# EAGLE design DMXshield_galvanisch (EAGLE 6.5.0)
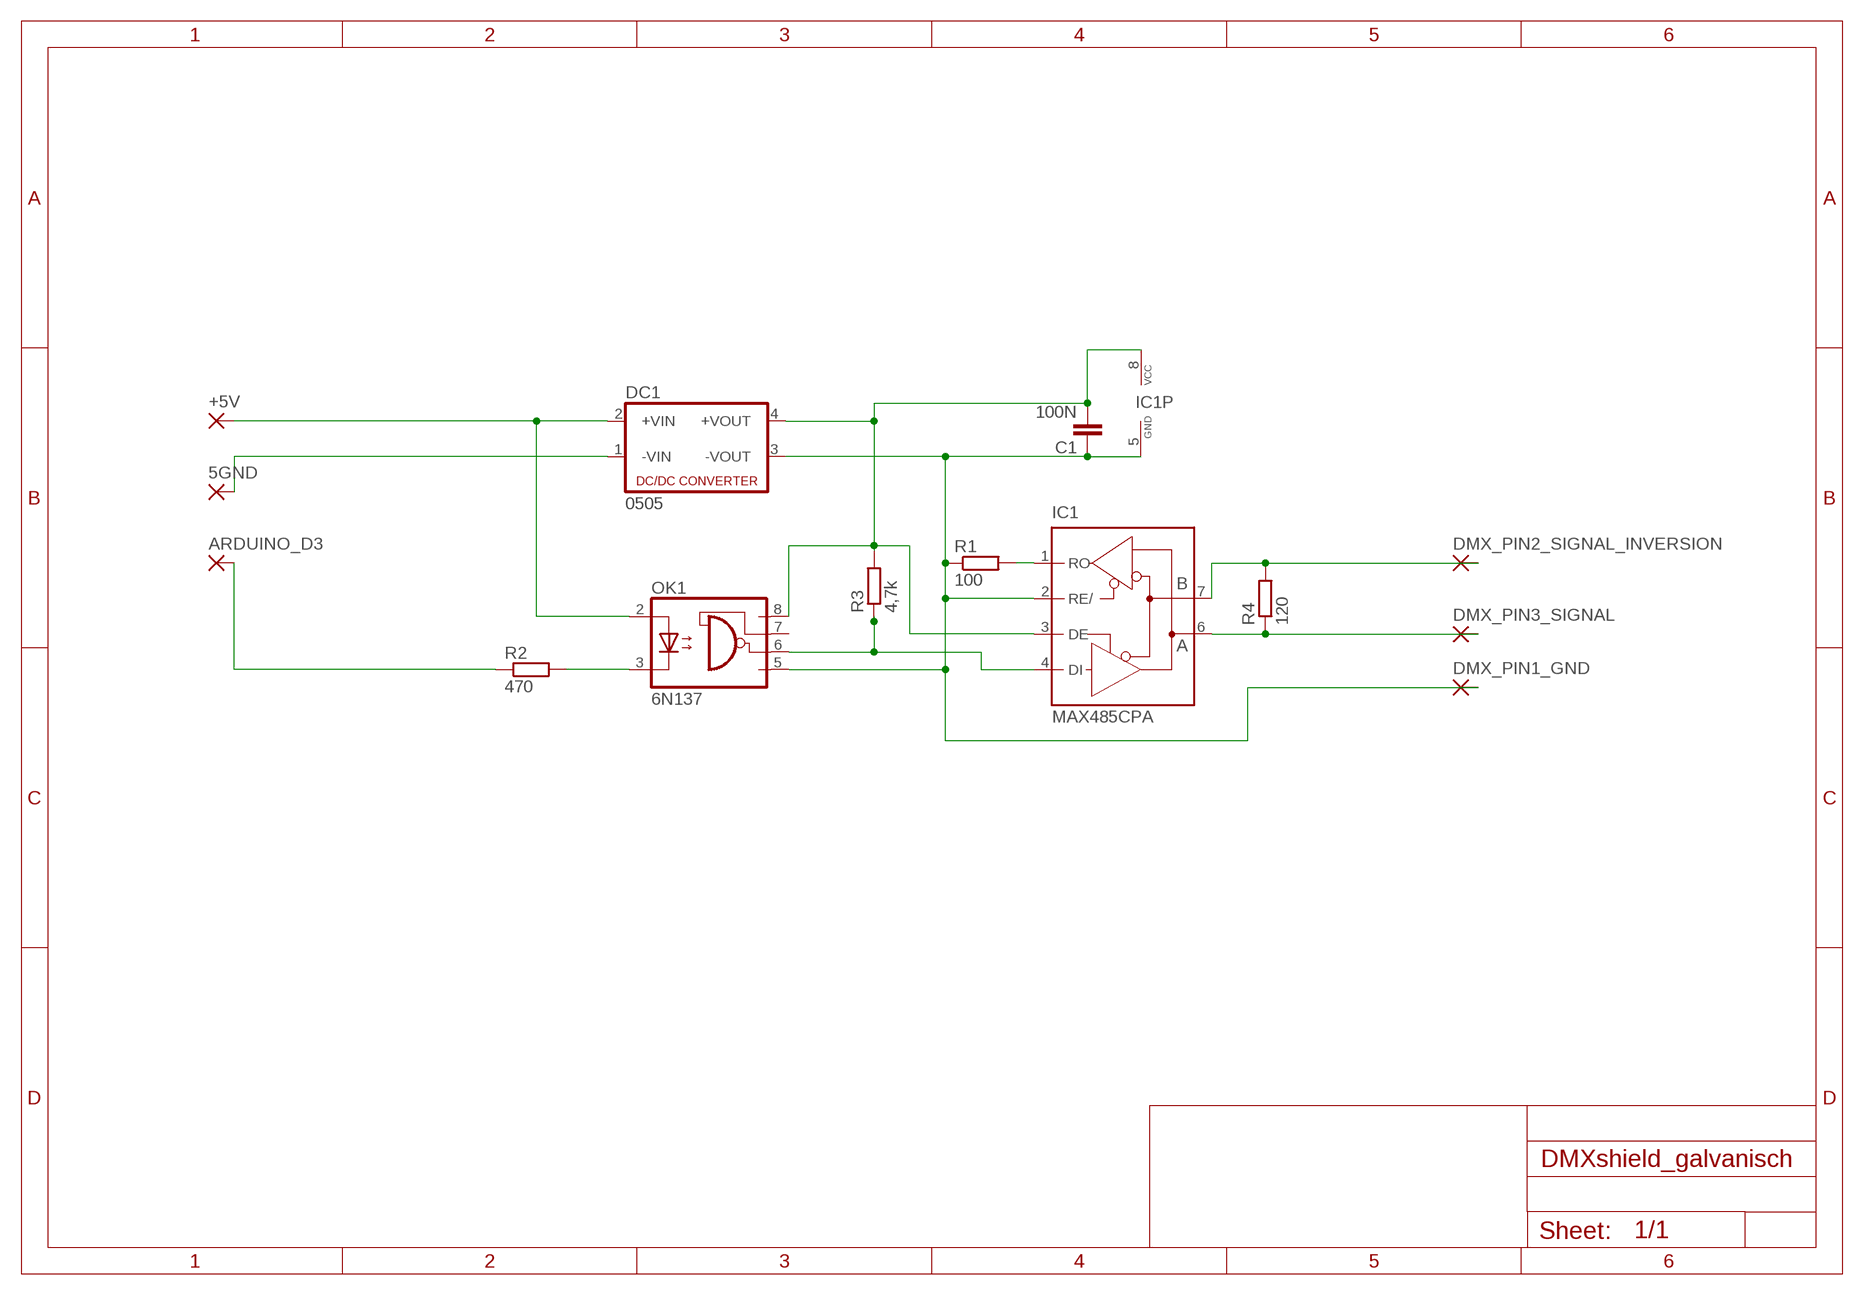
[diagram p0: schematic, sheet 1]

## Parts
5GND  3,81/1,4  [3,81/1,4]
+5V  3,81/1,4  [3,81/1,4]
ARDUINO_D3  3,81/1,4  [3,81/1,4]
C1  100N  C-EUC1206  [C1206]
DC1  0505  NME  [NME]
DMX_PIN1_GND  2,54/1,1  [2,54/1,1]
DMX_PIN2_SIGNAL_INVERSION  2,54/1,1  [2,54/1,1]
DMX_PIN3_SIGNAL  2,54/1,1  [2,54/1,1]
IC1  MAX485CPA  MAX481CPA  [DIL08]
OK1  6N137  [DIL08]
R1  100  R-EU_M1206  [M1206]
R2  470  R-EU_M1206  [M1206]
R3  4,7k  R-EU_M1206  [M1206]
R4  120  R-EU_M1206  [M1206]

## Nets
N$19: C1.2 DC1.4(+VOUT) IC1.3(DE) IC1.8(VCC) OK1.8(VCC) R3.2
N$21: +5V.1(P) DC1.2(+VIN) OK1.2(A)
N$32: IC1.1(RO) R1.2
N$33: 5GND.1(P) DC1.1(-VIN)
N$34: IC1.4(DI) OK1.6(VO) R3.1
N$35: ARDUINO_D3.1(P) R2.1
N$36: DMX_PIN3_SIGNAL.1(P) IC1.6(A) R4.1
N$37: DMX_PIN2_SIGNAL_INVERSION.1(P) IC1.7(B) R4.2
N$39: C1.1 DC1.3(-VOUT) DMX_PIN1_GND.1(P) IC1.2(RE/) IC1.5(GND) OK1.5(GND) R1.1
N$41: OK1.3(C) R2.2
Unconnected: OK1.7(VE)

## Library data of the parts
5GND +5V ARDUINO_D3 = wirepad:3,81/1,4: THROUGH-HOLE PAD
C1 = rcl:C-EU: CAPACITOR, European symbol
DC1 = dc-dc-converter:NME: DC-DC CONVERTER; MF: C & D TECHNOLOGIES, INC; MPN: NME1205D; OC_FARNELL: 1021466; OC_NEWARK: 98B8198
DMX_PIN1_GND DMX_PIN2_SIGNAL_INVERSION DMX_PIN3_SIGNAL = wirepad:2,54/1,1: THROUGH-HOLE PAD
IC1 = maxim:MAX481CPA: RS485 TRANSEIVER; MPN: MAX481CPA+; OC_FARNELL: unknown; OC_NEWARK: 99K3445
OK1 = optocoupler:6N137: MOTOROLA OPTO COUPLER; MPN: 6N137; OC_FARNELL: 1328376; OC_NEWARK: 52M1895
R1-R4 = rcl:R-EU_: RESISTOR, European symbol

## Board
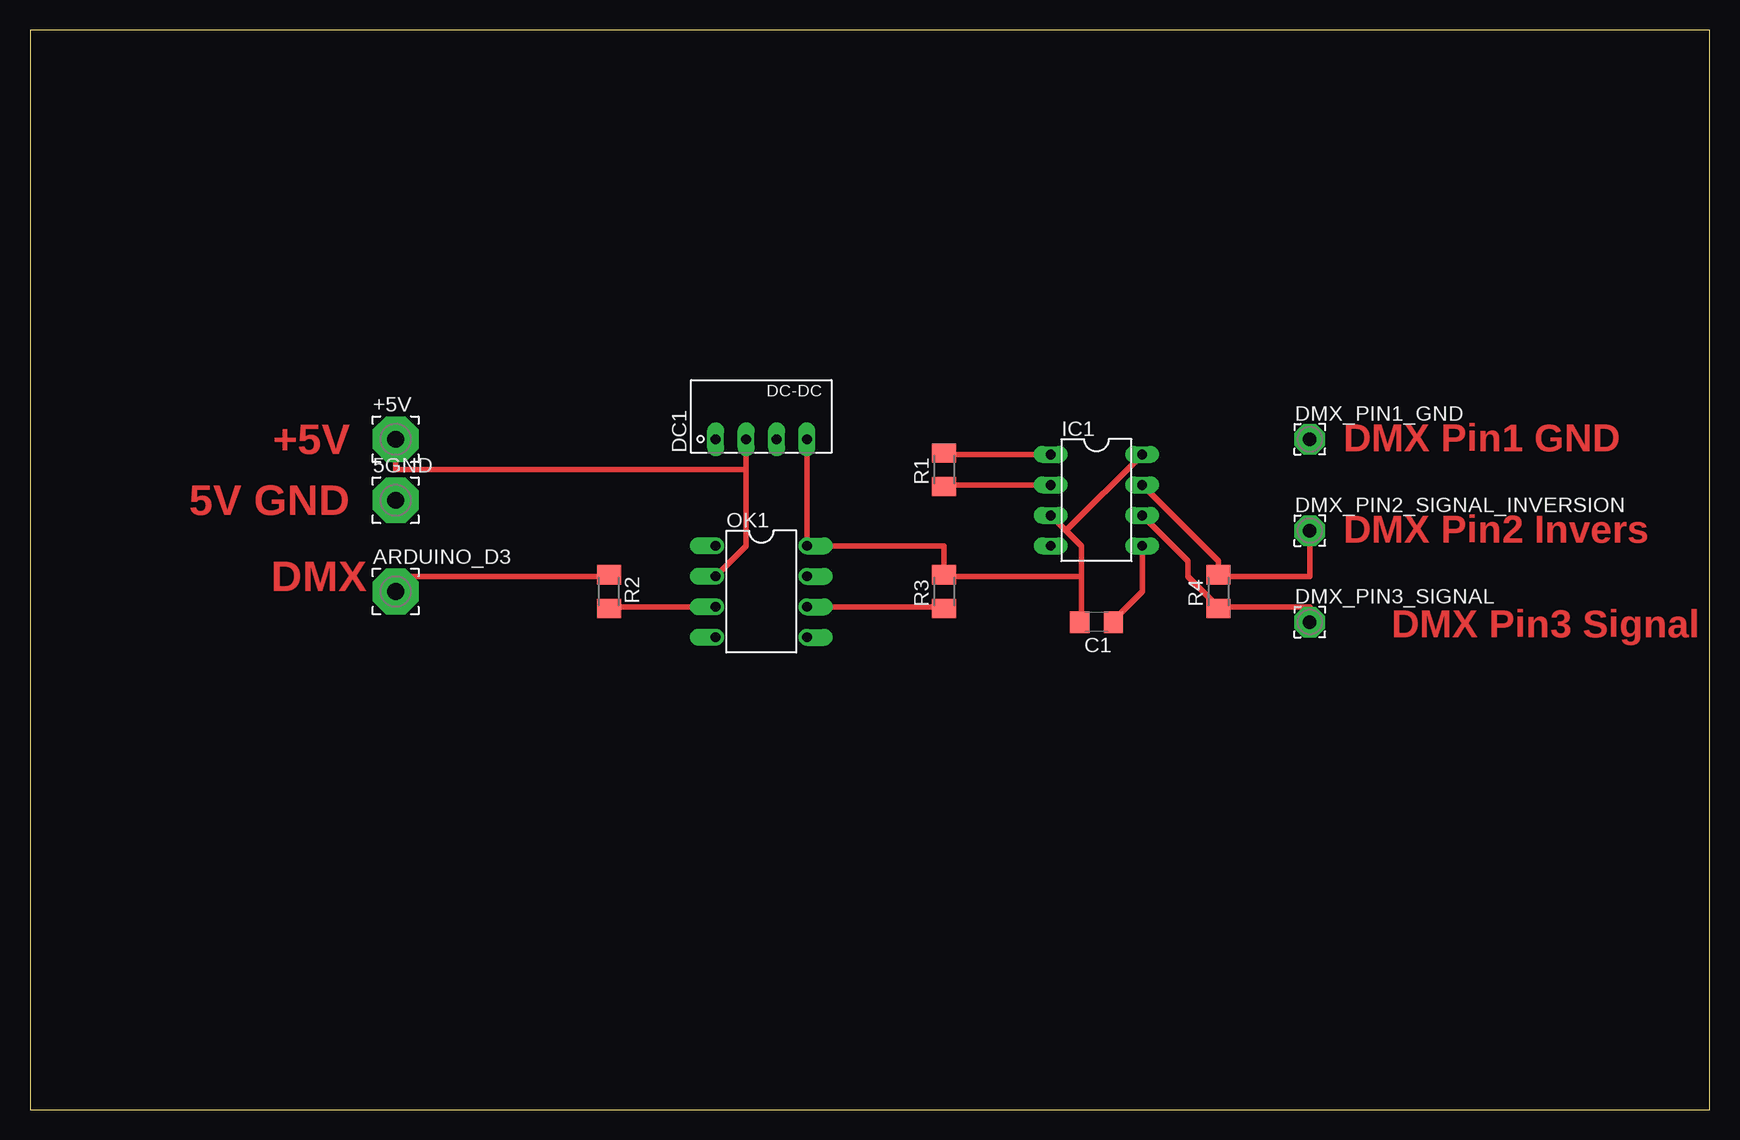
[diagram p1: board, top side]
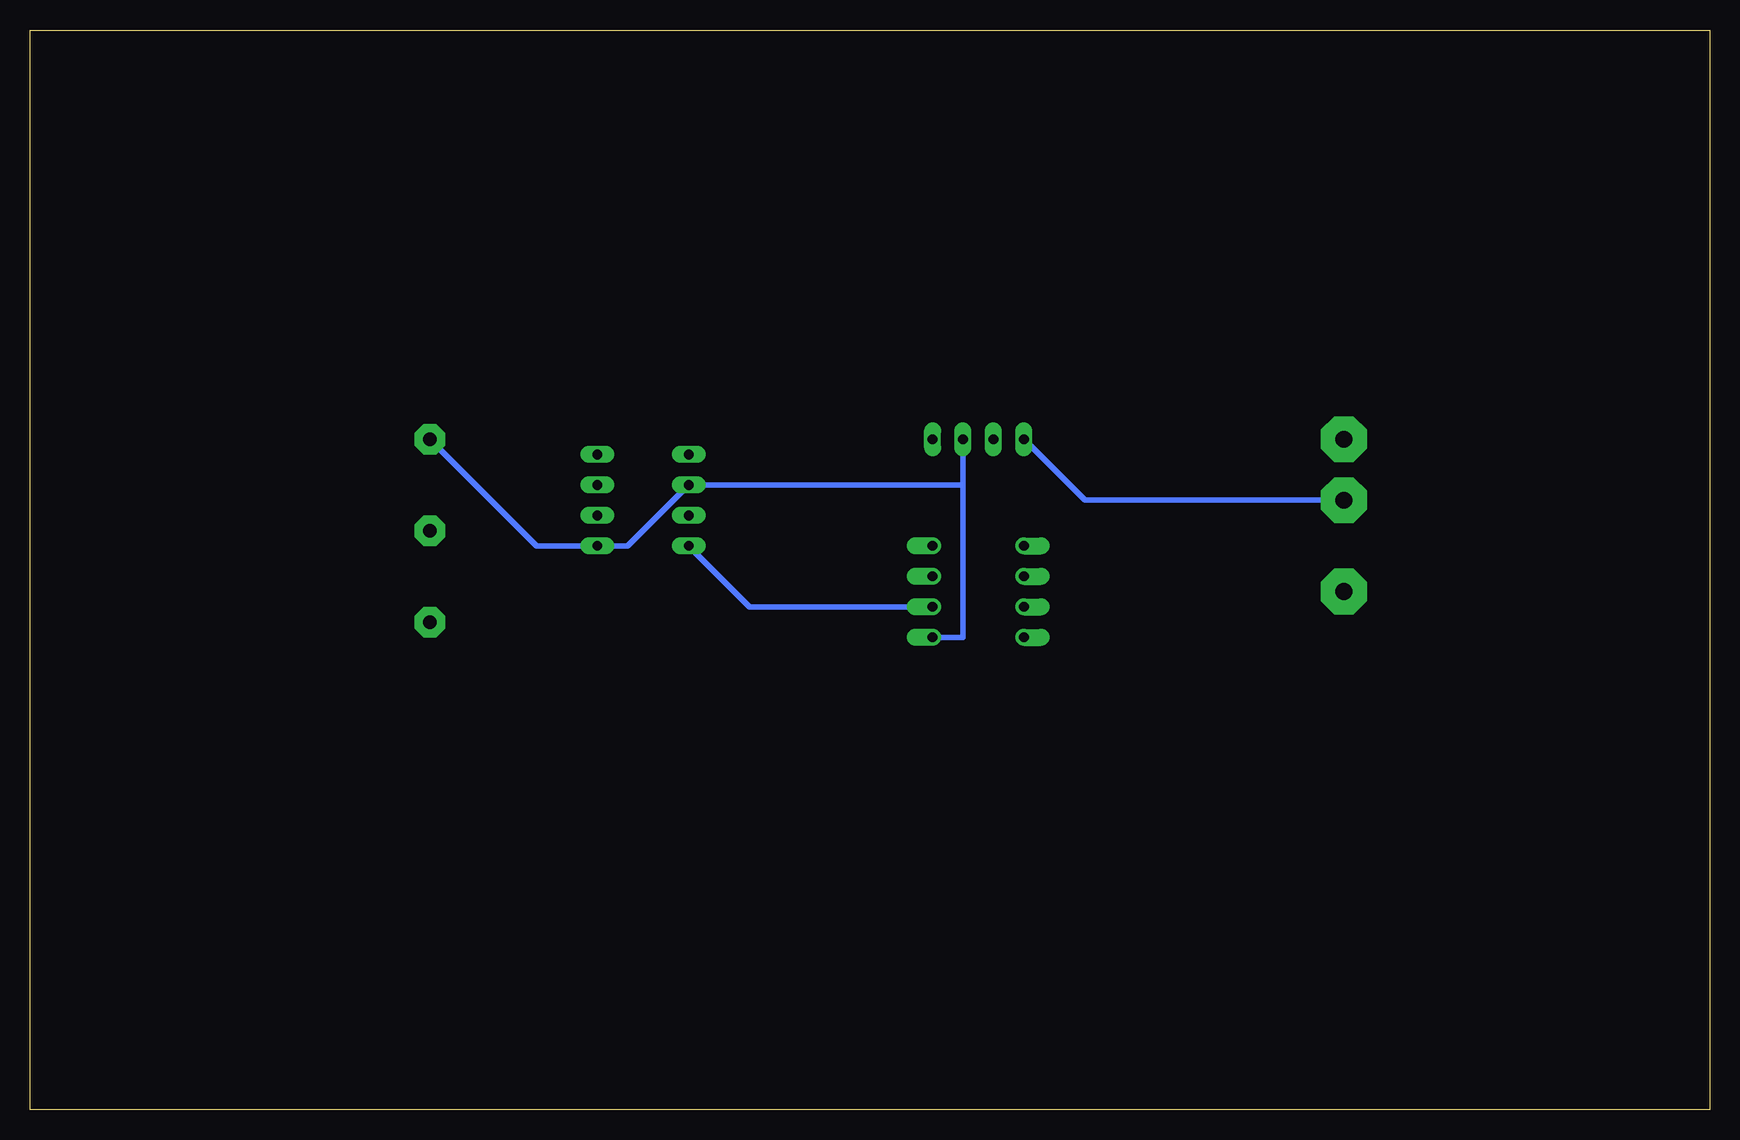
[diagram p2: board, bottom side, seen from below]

Size 140 x 90 mm. Coordinates in mm from the lower left corner, seen from the top.
Outline: 0,0 140,0 140,90 0,90 0,0
Copper layers (1*16): Top 0.035mm / dielectric 1.5mm / Bottom 0.035mm
Design rules "HTWG Sinnvoll *": minimum track width 18mil, minimum drill 0.4mm, track to track 12mil, track to pad 12mil, pad to pad 18mil, via to via 18mil, smd to smd 18mil, copper to edge 40mil, drill to drill 8mil, minimum pad ring 12mil, minimum via ring 20mil, stop-mask expansion 4mil, vias tented up to drill 0mil, thermal gap 10mil

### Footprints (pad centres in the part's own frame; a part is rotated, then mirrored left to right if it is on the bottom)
3,81/1,4 = drill 1.397 pad 3.81 octagon: 1 0,0
C1206 = smd 1.6 x 1.8: 1 -1.4,0; 2 1.4,0
NME = drill 0.813 long: 1 0,3.81; 2 0,1.27; 3 0,-1.27; 4 0,-3.81
2,54/1,1 = drill 1.118 pad 2.54 octagon: 1 0,0
DIL08 = drill 0.813 long: 1 -3.81,-3.81; 2 -1.27,-3.81; 3 1.27,-3.81; 4 3.81,-3.81; 5 3.81,3.81; 6 1.27,3.81; 7 -1.27,3.81; 8 -3.81,3.81
DIL08' = drill 0.813 offset: 1 -3.81,-3.81; 2 -1.27,-3.81; 3 1.27,-3.81; 4 3.81,-3.81; 5 3.81,3.81; 6 1.27,3.81; 7 -1.27,3.81; 8 -3.81,3.81
M1206 = smd 1.6 x 2: 1 -1.4,0; 2 1.4,0

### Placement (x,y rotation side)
5GND  30.48,50.8 0 top
+5V  30.48,55.88 0 top
ARDUINO_D3  30.48,43.18 0 top
C1  88.9,40.64 180 top
DC1  60.96,55.88 90 top
DMX_PIN1_GND  106.68,55.88 0 top
DMX_PIN2_SIGNAL_INVERSION  106.68,48.26 0 top
DMX_PIN3_SIGNAL  106.68,40.64 0 top
IC1  88.9,50.8 270 top
OK1  6N137  [DIL08']  60.96,43.18 270 top
R1  76.2,53.34 90 top
R2  48.26,43.18 270 top
R3  76.2,43.18 90 top
R4  99.06,43.18 90 top

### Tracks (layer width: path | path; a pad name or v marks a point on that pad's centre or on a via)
N$19
  Top 0.457: DC1.4 OK1.8 76.2,46.99 R3.2 76.2,44.45 87.63,44.45 | 87.63,44.45 87.63,46.99 86.36,48.26 | 87.63,44.45 87.63,40.64 C1.2 | IC1.3 86.36,48.26 | 86.36,48.26 IC1.8
N$21
  Top 0.457: OK1.2 59.69,46.99 59.69,53.34 | DC1.2 59.69,53.34 | 59.69,53.34 30.48,53.34 +5V.1
N$32
  Top 0.457: IC1.1 76.2,54.61 R1.2
N$33
  Bottom 0.457: DC1.1 52.07,50.8 5GND.1
N$34
  Top 0.457: OK1.6 76.2,41.91 R3.1
  Bottom 0.457: IC1.4 80.01,41.91 OK1.6
N$35
  Top 0.457: ARDUINO_D3.1 30.48,44.45 48.26,44.45 R2.1
N$36
  Top 0.457: 99.06,41.91 106.68,41.91 DMX_PIN3_SIGNAL.1 | IC1.6 96.52,45.72 96.52,44.45 99.06,41.91 | 99.06,41.91 R4.1
N$37
  Top 0.457: DMX_PIN2_SIGNAL_INVERSION.1 106.68,44.45 99.06,44.45 R4.2 99.06,45.72 IC1.7
N$39
  Top 0.457: IC1.2 76.2,52.07 R1.1 | IC1.5 92.71,43.18 90.17,40.64 C1.1
  Bottom 0.457: 62.23,52.07 62.23,39.37 OK1.5 | 62.23,52.07 DC1.3 | DMX_PIN1_GND.1 97.79,46.99 IC1.5 90.17,46.99 IC1.2 62.23,52.07
N$41
  Top 0.457: OK1.3 48.26,41.91 R2.2

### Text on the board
Top: +5V | DMX Pin1 GND | 5V GND | DMX Pin2 Invers | DMX | DMX Pin3 Signal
